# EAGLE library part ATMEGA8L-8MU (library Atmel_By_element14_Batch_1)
System Programmable Flash
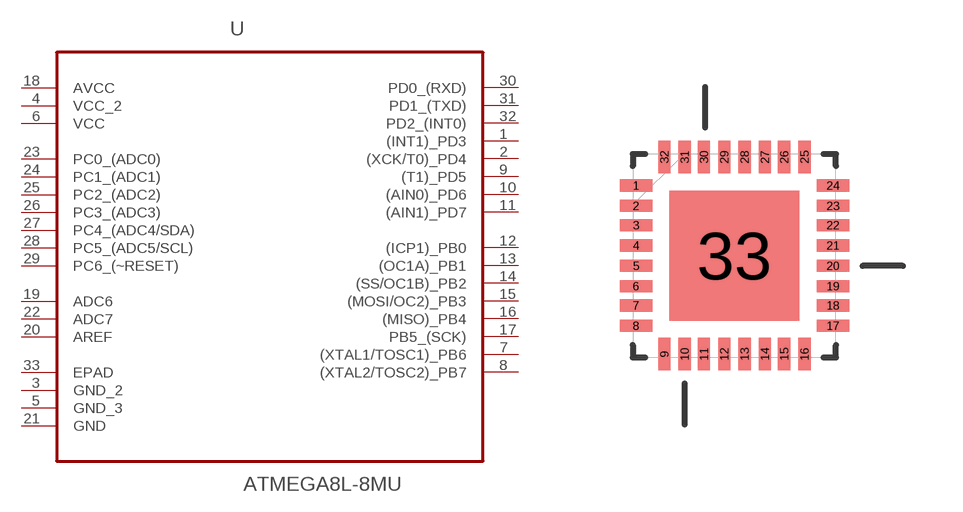
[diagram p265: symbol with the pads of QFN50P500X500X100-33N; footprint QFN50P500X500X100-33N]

Designator prefix U

## ATMEGA8L-8MU (DESCRIPTION: System Programmable Flash; MPN: ATMEGA8L-8MU; OC_FARNELL: 1455130; OC_NEWARK: 58M3751; PACKAGE: QFN-32; SUPPLIER: Atmel)  [QFN50P500X500X100-33N]
1  (INT1)_PD3
2  (XCK/T0)_PD4
3  GND_2  pas
4  VCC_2  pwr
5  GND_3  pas
6  VCC  pwr
7  (XTAL1/TOSC1)_PB6
8  (XTAL2/TOSC2)_PB7
9  (T1)_PD5
10  (AIN0)_PD6
11  (AIN1)_PD7
12  (ICP1)_PB0
13  (OC1A)_PB1
14  (SS/OC1B)_PB2
15  (MOSI/OC2)_PB3
16  (MISO)_PB4
17  PB5_(SCK)
18  AVCC  pwr
19  ADC6  in
20  AREF  in
21  GND  pas
22  ADC7  in
23  PC0_(ADC0)
24  PC1_(ADC1)
25  PC2_(ADC2)
26  PC3_(ADC3)
27  PC4_(ADC4/SDA)
28  PC5_(ADC5/SCL)
29  PC6_(~RESET)
30  PD0_(RXD)
31  PD1_(TXD)
32  PD2_(INT0)
33  EPAD  pas

## Footprint QFN50P500X500X100-33N (pad centres in mm)
smd 0.813 x 0.305: 1 -2.464,1.753; 2 -2.464,1.245; 3 -2.464,0.762; 4 -2.464,0.254; 5 -2.464,-0.254; 6 -2.464,-0.762; 7 -2.464,-1.245; 8 -2.464,-1.753; 17 2.464,-1.753; 18 2.464,-1.245; 19 2.464,-0.762; 20 2.464,-0.254; 21 2.464,0.254; 22 2.464,0.762; 23 2.464,1.245; 24 2.464,1.753
smd 0.305 x 0.813: 9 -1.753,-2.464; 10 -1.245,-2.464; 11 -0.762,-2.464; 12 -0.254,-2.464; 13 0.254,-2.464; 14 0.762,-2.464; 15 1.245,-2.464; 16 1.753,-2.464; 25 1.753,2.464; 26 1.245,2.464; 27 0.762,2.464; 28 0.254,2.464; 29 -0.254,2.464; 30 -0.762,2.464; 31 -1.245,2.464; 32 -1.753,2.464
smd 3.251 x 3.251: 33 0,0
